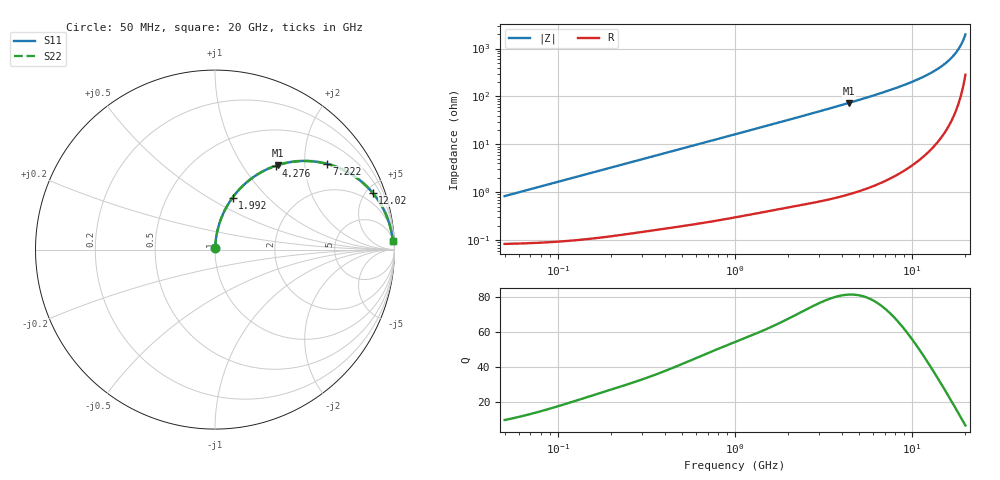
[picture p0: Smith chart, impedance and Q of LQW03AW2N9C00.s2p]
!Murata Part Number: LQW03AW2N9C00
!These Parameters are Measured in Series Mode Connection
!  o--[Z]--o
!Port1  Port2
!  o-------o
!Freq. Start=50[MHz] Stop=20[GHz], 401[Steps]
# Hz S RI R 50
!Freq.(Hz) S11(Real) S11(Imag) S21(Real) S21(Imag) S12(Real) S12(Imag) S22(Real) S22(Imag)
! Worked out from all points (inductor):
!   401 points, 50 MHz to 20 GHz, reference 50 ohm
!   read as one part in series: L = 2.63 nH near 51.52 MHz
!   highest Q = 81.1 at 4.406 GHz (marker M1), where L = 2.66 nH
!   S11 on the Smith chart (normalised r, x): 50 MHz: 1.00, +0.02; 1.992 GHz: 1.01, +0.65; 4.276 GHz: 1.02, +1.42; 7.222 GHz: 1.04, +2.59; 12.02 GHz: 1.13, +5.51; 20 GHz: 7, +39
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5e7  0.000903 0.00827  0.9991 -0.00827  0.9991 -0.00827  0.000903 0.00827
1.364002e8  0.00153 0.0225  0.9985 -0.0225  0.9985 -0.0225  0.00153 0.0225
3.721004e8  0.00533 0.0604  0.9947 -0.0604  0.9947 -0.0604  0.00533 0.0604
6.285508e8  0.0125 0.1007  0.9875 -0.1007  0.9875 -0.1007  0.0125 0.1007
1e9  0.0283 0.157  0.9717 -0.157  0.9717 -0.157  0.0283 0.157
1.454215e9  0.0558 0.2214  0.9442 -0.2214  0.9442 -0.2214  0.0558 0.2214
1.99176e9  0.0979 0.2898  0.9021 -0.2898  0.9021 -0.2898  0.0979 0.2898
2.728004e9  0.1683 0.3675  0.8317 -0.3675  0.8317 -0.3675  0.1683 0.3675
3.415248e9  0.2421 0.4221  0.7579 -0.4221  0.7579 -0.4221  0.2421 0.4221
4.275624e9  0.3382 0.467  0.6618 -0.467  0.6618 -0.467  0.3382 0.467
4.405649e9  0.3526 0.4717  0.6474 -0.4717  0.6474 -0.4717  0.3526 0.4717
5.683258e9  0.4877 0.4936  0.5123 -0.4936  0.5123 -0.4936  0.4877 0.4936
7.222371e9  0.6255 0.4771  0.3745 -0.4771  0.3745 -0.4771  0.6255 0.4771
7.442007e9  0.6426 0.4722  0.3574 -0.4722  0.3574 -0.4722  0.6426 0.4722
9.600142e9  0.7796 0.406  0.2204 -0.406  0.2204 -0.406  0.7796 0.406
1.201863e10  0.8782 0.3159  0.1218 -0.3159  0.1218 -0.3159  0.8782 0.3159
1.438523e10  0.9365 0.2286  0.0635 -0.2286  0.0635 -0.2286  0.9365 0.2286
1.550395e10  0.9548 0.1894  0.0452 -0.1894  0.0452 -0.1894  0.9548 0.1894
1.646126e10  0.9669 0.1573  0.0331 -0.1573  0.0331 -0.1573  0.9669 0.1573
1.747767e10  0.9767 0.1245  0.0233 -0.1245  0.0233 -0.1245  0.9767 0.1245
1.828096e10  0.9825 0.0997  0.0175 -0.0997  0.0175 -0.0997  0.9825 0.0997
2e10  0.9903 0.0493  0.00973 -0.0493  0.00973 -0.0493  0.9903 0.0493
